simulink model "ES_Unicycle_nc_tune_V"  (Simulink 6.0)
settings: Solver=ode3  StartTime=0.0  StopTime=tmax  FixedStep=deltaT  RelTol=1e-3
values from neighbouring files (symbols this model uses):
  a = 0.1    [ES_Unicycle_nc_values_tune_V.m]    (also in ES_Unicycle_nc_values_tune_V_moving.m = 0.04; ES_Unicycle_Values.m = 0.05; gradient2.m = 2*(df2 - df1); abs_perturbation.m = 0.01)
  c = 20    [ES_Unicycle_nc_values_tune_V.m]    (also in ES_Unicycle_nc_values_tune_V_moving.m = 50; abs_perturbation.m; abs_slidingmode.m; abs_steep.m = 1)
  centx = 0    [ES_Unicycle_nc_values_tune_V.m]    (also in ES_Unicycle_nc_values_tune_V_moving.m; ES_Unicycle_Values.m; ES_Unicycle_Values_SI.m = -1; ES_PointMass_Values.m = -1)
  centy = 0    [ES_Unicycle_nc_values_tune_V.m]    (also in ES_Unicycle_nc_values_tune_V_moving.m; ES_Unicycle_Values.m; ES_Unicycle_Values_SI.m = -1; ES_PointMass_Values.m = -1)
  h = 1    [ES_Unicycle_nc_values_tune_V.m]    (also in ES_Unicycle_nc_values_tune_V_moving.m; doublepointmass.m; pointmass.m)
  ICx = 2 - r    (= 1.8)    [ES_Unicycle_nc_values_tune_V.m]    (also in ES_Unicycle_nc_values_tune_V_moving.m = 1.5; ES_Unicycle_Values.m = 2; ES_Unicycle_Values_SI.m = 1; ES_PointMass_Values.m = 1)
  ICx_sen = 2    [ES_Unicycle_nc_values_tune_V.m]    (also in ES_Unicycle_nc_values_tune_V_moving.m)
  ICy = 2    [ES_Unicycle_nc_values_tune_V.m]    (also in ES_Unicycle_nc_values_tune_V_moving.m; ES_Unicycle_Values.m = 1; ES_Unicycle_Values_SI.m = 1; ES_PointMass_Values.m = 1)
  ICy_sen = 2    [ES_Unicycle_nc_values_tune_V.m]    (also in ES_Unicycle_nc_values_tune_V_moving.m)
  qx = 1/2    (= 0.5)    [ES_Unicycle_nc_values_tune_V.m]    (also in ES_Unicycle_nc_values_tune_V_moving.m; ES_PointMass_Values.m = 1; ES_SimplifyPointMass_Values.m = 1; ES_Unstable_Values.m = 1)
  qy = 1/4    (= 0.25)    [ES_Unicycle_nc_values_tune_V.m]    (also in ES_Unicycle_nc_values_tune_V_moving.m; ES_PointMass_Values.m = 0.5; ES_SimplifyPointMass_Values.m = 0.5; ES_Unstable_Values.m = 0.5)
  r = 0.2    [ES_Unicycle_nc_values_tune_V.m]    (also in ES_Unicycle_nc_values_tune_V_moving.m = 0.5; abs_trustregion.m = (f-mu(lambdar))/(f-M))
  w = 25    [ES_Unicycle_nc_values_tune_V.m]    (also in ES_Unicycle_nc_values_tune_V_moving.m; flnlesc_steep.m = 0.5; ionlesc_steep.m = 0.5; ltiesc_steep.m = 0.25)
  w1 = w/3    (= 8.33333333333)    [ES_Unicycle_nc_values_tune_V.m]    (also in ES_Unicycle_nc_values_tune_V_moving.m = 5; ltiesc_steep_derivatives_trackr.m = 2*pi/ts; ltiesc_steep_derivatives_trackr_constrained.m = 2*pi/ts; ltiesc_steep_derivatives_trackr_dac.m = 2*pi/ts)
libraries: simulink x2

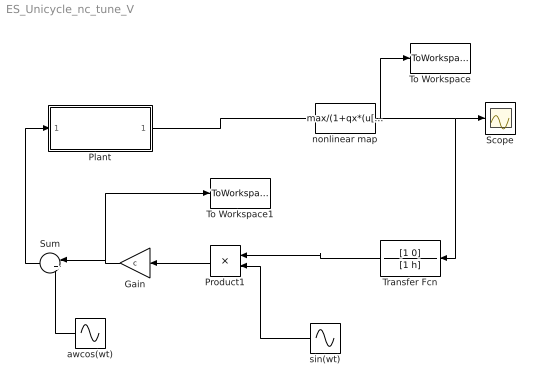
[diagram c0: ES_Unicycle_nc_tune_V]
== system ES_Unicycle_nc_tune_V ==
  Gain : Gain  Orientation=left  Gain=c
  Plant : Subsystem
  Product1 : Product  Orientation=left
  Scope : Scope
  Sum : Sum  Orientation=left  Inputs=|++
  To Workspace : ToWorkspace  VariableName=f  SampleTime=-1  SaveFormat=Array
  To Workspace1 : ToWorkspace  VariableName=v  SampleTime=-1  SaveFormat=Array
  Transfer Fcn : TransferFcn  Orientation=left  Numerator=[1 0]  Denominator=[1 h]
  awcos(wt) : Sin  Orientation=left  Amplitude=a*w  Frequency=w  Phase=pi/2  SampleTime=0
  nonlinear map : Fcn  Expr=max/(1+qx*(u[1]-centx)^2+qy*(u[2]-centy)^2)
  sin(wt) : Sin  Orientation=left  Frequency=w  SampleTime=0
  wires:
  nonlinear map/1 -> Transfer Fcn/1, Scope/1, To Workspace/1
  sin(wt)/1 -> Product1/2
  Transfer Fcn/1 -> Product1/1
  Product1/1 -> Gain/1
  Gain/1 -> Sum/1, To Workspace1/1
  awcos(wt)/1 -> Sum/2
  Plant/1(Out1) -> nonlinear map/1
  Sum/1 -> Plant/1(In1)

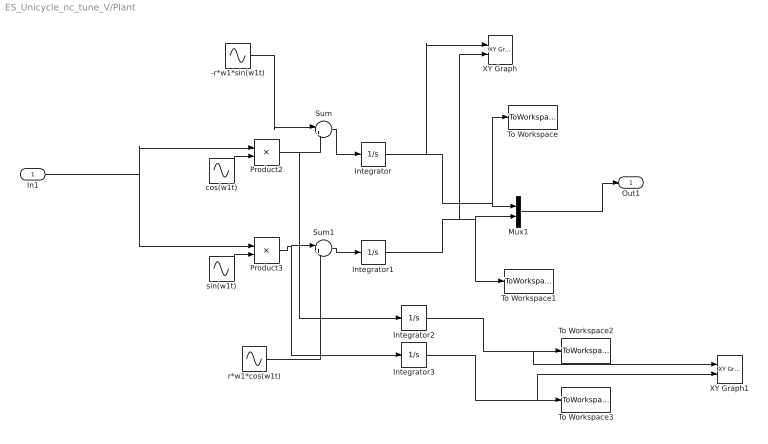
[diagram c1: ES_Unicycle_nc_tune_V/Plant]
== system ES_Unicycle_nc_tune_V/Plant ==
  In1 : Inport  Port=1  LatchInput=off
  -r*w1*sin(w1t) : Sin  Amplitude=-r*w1  Frequency=w1  SampleTime=0
  Integrator : Integrator  InitialCondition=ICx_sen
  Integrator1 : Integrator  InitialCondition=ICy_sen
  Integrator2 : Integrator  InitialCondition=ICx
  Integrator3 : Integrator  InitialCondition=ICy
  Mux1 : Mux  Inputs=2
  Product2 : Product
  Product3 : Product
  Sum : Sum  Inputs=|++
  Sum1 : Sum  Inputs=|++
  To Workspace : ToWorkspace  VariableName=x_sen  SampleTime=-1  SaveFormat=Array
  To Workspace1 : ToWorkspace  VariableName=y_sen  SampleTime=-1  SaveFormat=Array
  To Workspace2 : ToWorkspace  VariableName=x  SampleTime=-1  SaveFormat=Array
  To Workspace3 : ToWorkspace  VariableName=y  SampleTime=-1  SaveFormat=Array
  XY Graph : simulink/Sinks/XY Graph  xmin=-1  xmax=2  ymin=-1  ymax=2  st=-1
  XY Graph1 : simulink/Sinks/XY Graph  xmin=-1  xmax=2  ymin=-1  ymax=2  st=-1
  cos(w1t) : Sin  Frequency=w1  Phase=pi/2+.3  SampleTime=0
  r*w1*cos(w1t) : Sin  Amplitude=r*w1  Frequency=w1  Phase=pi/2  SampleTime=0
  sin(w1t) : Sin  Frequency=w1  Phase=.3  SampleTime=0
  Out1 : Outport
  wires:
  cos(w1t)/1 -> Product2/2
  sin(w1t)/1 -> Product3/2
  In1/1 -> Product2/1, Product3/1
  Mux1/1 -> Out1/1
  Integrator/1 -> Mux1/1, To Workspace/1, XY Graph/1
  Integrator1/1 -> Mux1/2, To Workspace1/1, XY Graph/2
  Product3/1 -> Sum1/1, Integrator3/1
  Sum1/1 -> Integrator1/1
  Product2/1 -> Sum/2, Integrator2/1
  Sum/1 -> Integrator/1
  -r*w1*sin(w1t)/1 -> Sum/1
  r*w1*cos(w1t)/1 -> Sum1/2
  Integrator2/1 -> To Workspace2/1, XY Graph1/1
  Integrator3/1 -> To Workspace3/1, XY Graph1/2
